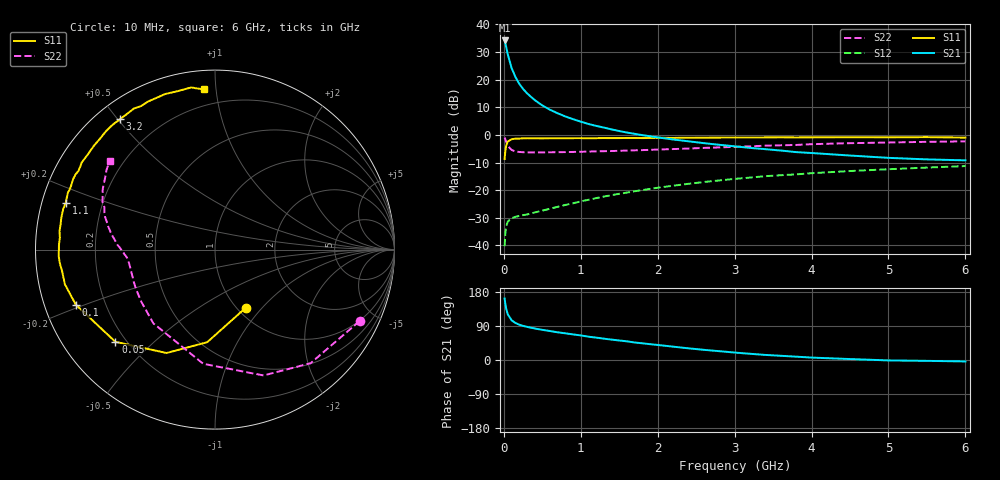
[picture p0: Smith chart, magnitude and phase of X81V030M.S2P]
! SIEMENS Small Signal Semiconductors
! BFP136W
! Si NPN RF Bipolar Junction Transistor in SOT343
! VCE = 1 V  IC = 30 mA
! Common Emitter S-Parameters:  September  1994
# GHz  S  MA  R  50
!  f  S11  S21  S12  S22
! GHz  MAG  ANG  MAG  ANG  MAG  ANG  MAG  ANG
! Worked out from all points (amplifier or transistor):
!   40 points, 10 MHz to 6 GHz, reference 50 ohm
!   highest |S21| = 34.2 dB at 10 MHz (marker M1)
!   |S21| within 3 dB of that: start of sweep to 35.32 MHz
!   unconditionally stable (mu >= 1): 688.3 MHz to 2.935 GHz; 3.786 GHz to 3.818 GHz; 5.828 GHz to end of sweep
!   at 200 MHz: K = 0.45, MSG = 23.9 dB, |S12| = -29.3 dB
!   at 1.5 GHz: K = 1.16, MAG = 9.0 dB, |S12| = -21.3 dB
!   at 6 GHz: K = 1.02, MAG = 0.1 dB, |S12| = -11.3 dB
!   S11 on the Smith chart (normalised r, x): 10 MHz: 1.09, -0.82; 50 MHz: 0.16, -0.38; 100 MHz: 0.09, -0.19; 1.1 GHz: 0.07, +0.15; 3.2 GHz: 0.07, +0.51; 6 GHz: 0.10, +0.93
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0.01  0.3668 -62.3  51.34 162.5  0.0097 71.3  0.8988 -26.3
0.02  0.5177 -94.8  45.35 147.4  0.0168 59.3  0.8273 -49.9
0.03  0.6362 -115.1  39.42 136.0  0.022 49.7  0.7516 -68.9
0.05  0.7563 -137.2  29.03 121.1  0.0269 36.7  0.6396 -95.9
0.1  0.834 -158.4  16.43 105.0  0.0313 26.7  0.5355 -129.9
0.15  0.8585 -167.0  11.22 97.7  0.0329 25.4  0.5027 -145.0
0.2  0.8599 -171.7  8.444 93.3  0.0343 26.3  0.4919 -153.3
0.25  0.8681 -175.1  6.818 90.0  0.0354 27.6  0.487 -158.5
0.3  0.8714 -177.5  5.697 87.6  0.0363 29.3  0.4834 -162.0
0.4  0.8698 178.4  4.292 83.2  0.0395 34.0  0.4829 -166.5
0.5  0.8669 175.5  3.422 79.6  0.0426 37.4  0.4835 -169.4
0.6  0.8721 173.4  2.858 76.5  0.0462 40.6  0.4851 -171.3
0.7  0.8717 170.7  2.464 73.1  0.05 43.7  0.4873 -172.5
0.8  0.8738 169.0  2.16 70.4  0.0541 45.9  0.4895 -173.7
1.1  0.8714 162.5  1.579 61.5  0.0671 49.9  0.5002 -176.3
1.4  0.8758 157.4  1.261 53.8  0.0814 52.2  0.5117 -178.4
1.6  0.8825 153.6  1.106 49.3  0.0905 52.7  0.5215 -179.9
2.2  0.8849 143.3  0.828 35.2  0.1204 51.2  0.555 175.4
3.2  0.8988 126.0  0.583 16.4  0.1692 44.1  0.6224 165.6
4.5  0.9102 107.8  0.424 2.5  0.2222 32.5  0.7099 151.8
5.5  0.9132 98.4  0.361 -2.3  0.2568 24.5  0.7508 143.5
6  0.8946 94.1  0.347 -3.8  0.2735 20.0  0.7655 140.1
